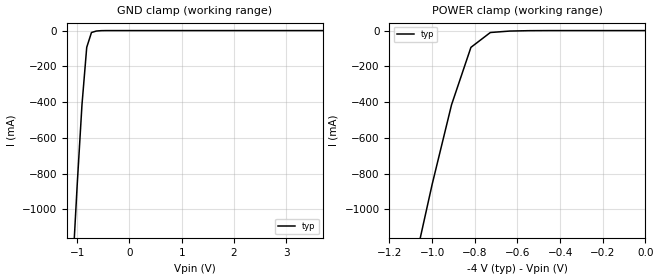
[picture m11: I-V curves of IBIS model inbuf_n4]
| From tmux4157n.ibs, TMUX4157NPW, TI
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| inbuf_n4
[Model]   inbuf_n4
Model_type   Input
Vinl = 0.8
Vinh = 1.35
|   typ   min   max
C_comp   6.976543e-12   NA   NA
[Voltage Range]   -4   NA   NA
[Temperature Range]   27   NA   NA
[Power Clamp Reference]   -4   NA   NA
[GND Clamp Reference]   0   NA   NA
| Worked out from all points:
|   GND clamp passes 1 mA (typ) near -0.57 V on its own axis
|   POWER clamp passes 1 mA (typ) near -0.57 V on its own axis
[GND Clamp]
|   Voltage   I(typ)   I(min)   I(max)
-4V       -15.02A    NA         NA
-1.091V   -1.348A    NA         NA
-1V       -859.5mA   NA         NA
-909.1mV  -414.9mA   NA         NA
-818.2mV  -93.75mA   NA         NA
-727.3mV  -10.84mA   NA         NA
-636.4mV  -2.673mA   NA         NA
-454.5mV  -36.19uA   NA         NA
5V        1.753uA    NA         NA
[POWER Clamp]
|   Voltage   I(typ)   I(min)   I(max)
-9V       -34.16A    NA         NA
-1.091V   -1.348A    NA         NA
-1V       -859.8mA   NA         NA
-909.1mV  -414.9mA   NA         NA
-818.2mV  -93.76mA   NA         NA
-727.3mV  -10.84mA   NA         NA
-545.5mV  -482.9uA   NA         NA
0V        93.38pA    NA         NA
